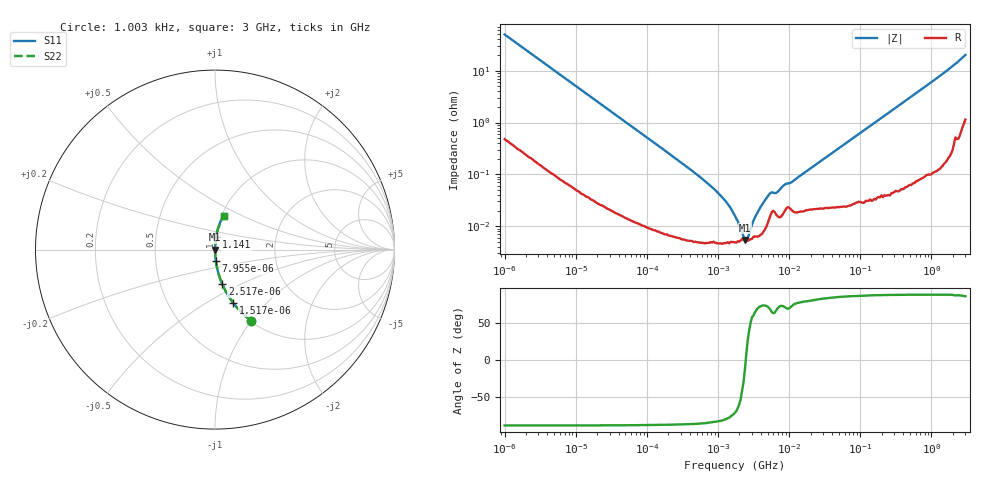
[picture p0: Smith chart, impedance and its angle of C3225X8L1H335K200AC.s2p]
! S-Parameter Data Generated by TDK Corporation
! Copyright(C) 2022 TDK Corporation.
! All Rights Reserved.
! TDK P/N: C3225X8L1H335K200AC (Multilayer Ceramic Chip Capacitor)
! Property: C=3.3uF
! Size(LxWxT): 3.2x2.5x2mm
! Model Type: s2p (Touchstone File Format Version 1.0)
! Frequency: DC=Yes Start=0.00100273MHz Stop=3000MHz 326points Log-sweep
! Model Generated on Apr. 15, 2022
! Port Assignments:
!  1 ---| |--- 2
! Applicable Conditions:
!  Temperature = 25 degC
!  DC Bias Voltage = 0 V
!  Small Signal Operation
! Terms and conditions regarding TDK Simulation Models
! (1)This simulation model is being provided solely for informational purposes. Please refer to the specifications of the products in terms of detailed characteristics of such products.
! (2)In no event shall TDK Corporation of any of its subsidiaries be liable for any loss or damage arising, directly or indirectly,
!  From any information contained in this simulation model, including, but not limited to loss or damages arising from any inaccuracies, omissions or errors in connection with such information.
! (3)Any and all copyrights on this simulation model are owned by TDK Corporation.
!  Duplication or redistribution of this simulation model without prior written permission from TDK Corporation is prohibited.
! (4)This simulation model is subject to any modification or change without any prior notice.
! (5)Neither TDK Corporation nor any of its subsidiaries shall make any warranty, express or implied,
!  Including but not limited to the correctness, implied warranties of merchantability and fitness for a particular purpose with respect to this simulation models.
! (6)The use of this simulation model shall be deemed to have consented to the terms and conditions hereof.
# Hz S MA R 50
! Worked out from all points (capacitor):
!   325 points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, 1.003 kHz to 3 GHz, reference 50 ohm
!   read as one part in series: C = 3.17 uF near 1.05 kHz
!   lowest |Z| = 5.44 mohm at 2.394 MHz (marker M1)
!   series resonance near 2.459 MHz, so ESL is about 1.3 nH
!   S11 on the Smith chart (normalised r, x): 1.003 kHz: 1.01, -1.00; 1.517 kHz: 1.01, -0.66; 2.517 kHz: 1.00, -0.40; 7.955 kHz: 1.00, -0.13; 1.141 GHz: 1.00, +0.14; 3 GHz: 1.02, +0.40
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1002.73  0.4451 -63.0  0.8912 26.4  0.8912 26.4  0.4451 -63.0
1517.29  0.3135 -71.2  0.9467 18.3  0.9467 18.3  0.3135 -71.2
2517.28  0.1962 -78.1  0.9787 11.3  0.9787 11.3  0.1962 -78.1
7954.6  0.0638 -85.8  0.9973 3.7  0.9973 3.7  0.0638 -85.8
12036.7  0.04233 -87.0  0.9987 2.4  0.9987 2.4  0.04233 -87.0
151292  0.00342 -88.5  0.9999 0.2  0.9999 0.2  0.00342 -88.5
869641  0.0005315 -84.5  0.9999 0.0  0.9999 0.0  0.0005315 -84.5
1315910  0.0002888 -80.5  1 0.0  1 0.0  0.0002888 -80.5
1816100  0.000139 -69.6  1 0.0  1 0.0  0.000139 -69.6
1991200  0.000103 -60.6  0.9999 0.0  0.9999 0.0  0.000103 -60.6
2393670  5.439e-05 -12.3  0.9999 0.0  0.9999 0.0  5.439e-05 -12.3
2877490  8.925e-05 51.1  0.9999 -0.0  0.9999 -0.0  8.925e-05 51.1
3013020  0.0001083 58.2  0.9999 -0.0  0.9999 -0.0  0.0001083 58.2
3971240  0.0002353 73.1  0.9999 -0.0  0.9999 -0.0  0.0002353 73.1
5480730  0.000439 68.1  0.9998 -0.0  0.9998 -0.0  0.000439 68.1
6588530  0.0004401 67.7  0.9998 -0.0  0.9998 -0.0  0.0004401 67.7
8683870  0.0006356 71.9  0.9998 -0.0  0.9998 -0.0  0.0006356 71.9
1.09308e7  0.0007112 73.5  0.9998 -0.0  0.9998 -0.0  0.0007112 73.5
2.18003e7  0.001418 81.3  0.9998 -0.1  0.9998 -0.1  0.001418 81.3
2.61689e8  0.0161 87.7  0.9995 -0.9  0.9995 -0.9  0.0161 87.7
1.14126e9  0.0685 85.1  0.9965 -3.9  0.9965 -3.9  0.0685 85.1
3e9  0.1952 75.5  0.9698 -11.2  0.9698 -11.2  0.1952 75.5
